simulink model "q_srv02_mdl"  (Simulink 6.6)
settings: Solver=ode1  StartTime=0.0  StopTime=inf  FixedStep=0.002  RelTol=1e-3  AbsTol=1e-6
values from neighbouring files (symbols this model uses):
  K = Am / Beq_v    [d_model_param.m]    (also in setup_srv02_exp01_mdl.m = 1)
  K_AMP = 1    [setup_srv02_exp01_mdl.m]    (also in setup_srv02_exp02_pos.m; setup_srv02_exp03_spd.m)
  K_ENC = 0    [config_srv02.m]
  K_POT = -(352 * pi / 180 / 10)    (= -0.614355896702)    [config_srv02.m]
  K_TACH = -(1000 * 2 * pi / 60 / 1.5 / Kg)    [config_srv02.m]
  tau = Jeq / Beq_v    [d_model_param.m]    (also in setup_srv02_exp01_mdl.m = 0.1)
  VMAX_AMP = 0    [config_srv02.m]
  VMAX_DAC = 10    [setup_srv02_exp01_mdl.m]    (also in setup_srv02_exp02_pos.m; setup_srv02_exp03_spd.m)
  wcf_e = 2 * pi * 25.0    (= 157.079632679)    [setup_srv02_exp01_mdl.m]    (also in setup_srv02_exp02_pos.m = 314.159265359; setup_srv02_exp03_spd.m = 395.840674352)
  zetaf_e = 0.9    [setup_srv02_exp01_mdl.m]    (also in setup_srv02_exp02_pos.m; setup_srv02_exp03_spd.m)
undefined symbols (not defined in the file or in its folder): HIL, qc_get_step_size
libraries: quarc_library x5, simulink x2

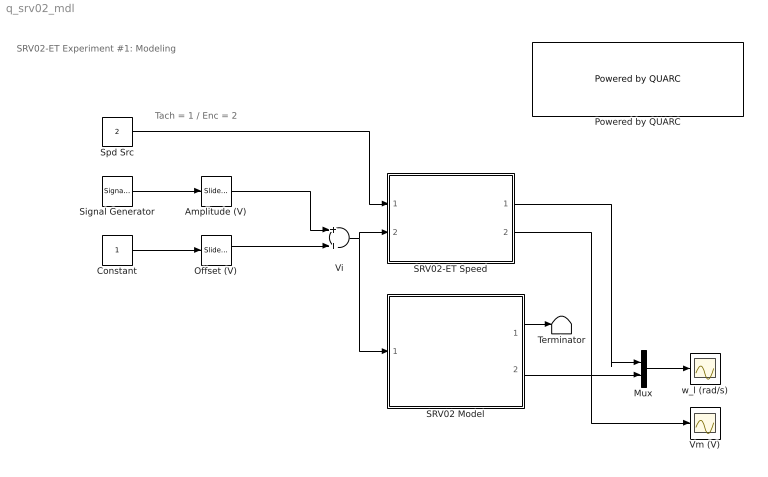
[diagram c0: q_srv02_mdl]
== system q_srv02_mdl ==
  note: SRV02-ET Experiment #1: Modeling
  note: Tach = 1 / Enc = 2
  Amplitude (V) : simulink/Math Operations/Slider Gain  SystemSampleTime=-1  low=0  gain=1  high=5
  Constant : Constant
  Mux : Mux  Inputs=2
  Offset (V) : simulink/Math Operations/Slider Gain  SystemSampleTime=-1  low=-5  gain=1.5  high=5
  Powered by QUARC : quarc_library/Logos/Powered by QUARC  SystemSampleTime=-1
  SRV02 Model : Subsystem
  SRV02-ET Speed : Subsystem
  Signal Generator : SignalGenerator  WaveForm=square  Frequency=0.4
  Spd Src : Constant  Value=2
  Terminator : Terminator
  Vi : Sum  OutScaling=2^-10
  Vm (V) : Scope
  w_l (rad/s) : Scope
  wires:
  Constant/1 -> Offset (V)/1
  Offset (V)/1 -> Vi/2
  Vi/1 -> SRV02 Model/1(Vi (V)), SRV02-ET Speed/2(Vi (V))
  Mux/1 -> w_l (rad/s)/1
  SRV02-ET Speed/2(Vm (V)) -> Vm (V)/1
  SRV02 Model/2(omega_l (rad/s)) -> Mux/2
  SRV02-ET Speed/1(omega_l (rad/s)) -> Mux/1
  SRV02 Model/1(theta_l (rad)) -> Terminator/1
  Signal Generator/1 -> Amplitude (V)/1
  Amplitude (V)/1 -> Vi/1
  Spd Src/1 -> SRV02-ET Speed/1(spd src)

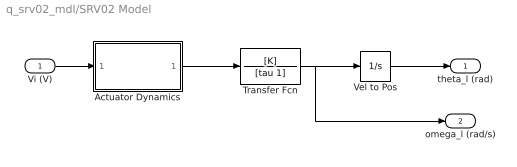
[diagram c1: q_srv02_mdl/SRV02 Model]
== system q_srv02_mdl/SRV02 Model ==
  Vi (V) : Inport
  Actuator Dynamics : Subsystem
  Transfer Fcn : TransferFcn  Numerator=[K]  Denominator=[tau 1]
  Vel to Pos : Integrator
  theta_l (rad) : Outport
  omega_l (rad/s) : Outport  Port=2
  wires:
  Vi (V)/1 -> Actuator Dynamics/1(Vi (V))
  Actuator Dynamics/1(Vm (V)) -> Transfer Fcn/1
  Vel to Pos/1 -> theta_l (rad)/1
  Transfer Fcn/1 -> Vel to Pos/1, omega_l (rad/s)/1

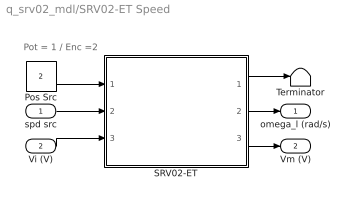
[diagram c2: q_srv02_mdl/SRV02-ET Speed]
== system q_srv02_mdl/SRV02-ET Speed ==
  note: Pot = 1 / Enc =2
  spd src : Inport
  Vi (V) : Inport  Port=2
  Pos Src : Constant  Value=2
  SRV02-ET : Subsystem
  Terminator : Terminator
  omega_l (rad/s) : Outport
  Vm (V) : Outport  Port=2
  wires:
  SRV02-ET/3(Vm (V)) -> Vm (V)/1
  Vi (V)/1 -> SRV02-ET/3(Vi (V))
  SRV02-ET/2(omega_l (rad/s)) -> omega_l (rad/s)/1
  spd src/1 -> SRV02-ET/2(spd src)
  SRV02-ET/1(theta_l (rad)) -> Terminator/1
  Pos Src/1 -> SRV02-ET/1(pos src)

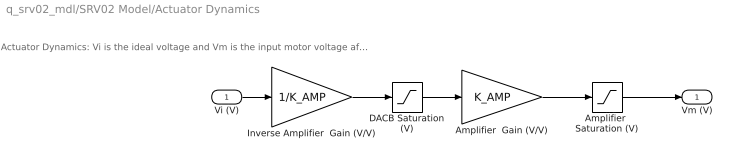
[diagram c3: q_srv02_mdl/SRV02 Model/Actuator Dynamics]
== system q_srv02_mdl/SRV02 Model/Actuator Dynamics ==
  note: Actuator Dynamics: Vi is the ideal voltage and Vm is the input motor voltage after going through the DACB and amplifier limitiations.
  Vi (V) : Inport
  Amplifier  Gain (V/V) : Gain  Gain=K_AMP
  Amplifier  Saturation (V) : Saturate  UpperLimit=VMAX_AMP  LowerLimit=-VMAX_AMP
  DACB Saturation (V) : Saturate  UpperLimit=VMAX_DAC  LowerLimit=-VMAX_DAC
  Inverse Amplifier  Gain (V/V) : Gain  Gain=1/K_AMP
  Vm (V) : Outport
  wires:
  Inverse Amplifier  Gain (V/V)/1 -> DACB Saturation (V)/1
  DACB Saturation (V)/1 -> Amplifier  Gain (V/V)/1
  Amplifier  Gain (V/V)/1 -> Amplifier  Saturation (V)/1
  Vi (V)/1 -> Inverse Amplifier  Gain (V/V)/1
  Amplifier  Saturation (V)/1 -> Vm (V)/1

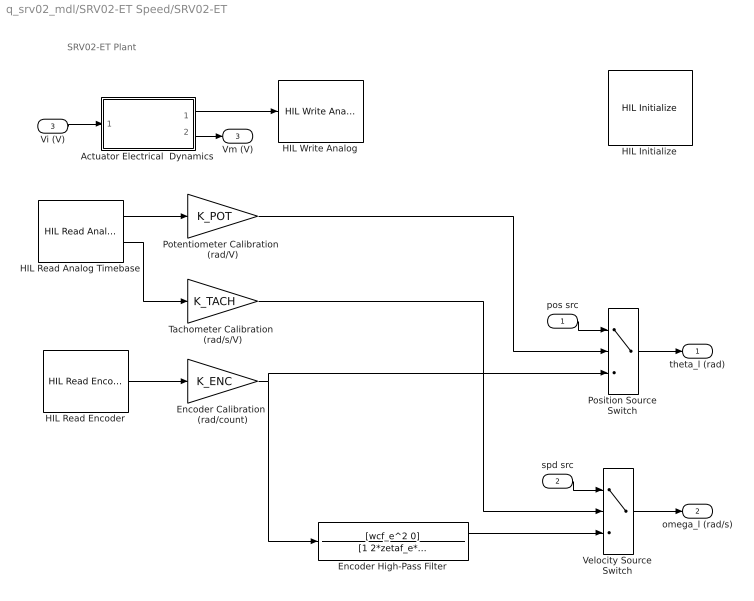
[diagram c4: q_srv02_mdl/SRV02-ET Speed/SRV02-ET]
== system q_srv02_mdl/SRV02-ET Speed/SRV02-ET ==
  note: SRV02-ET Plant
  pos src : Inport
  spd src : Inport  Port=2
  Vi (V) : Inport  Port=3
  Actuator Electrical  Dynamics : Subsystem
  Encoder Calibration  (rad/count) : Gain  Gain=K_ENC
  Encoder High-Pass Filter : TransferFcn  Numerator=[wcf_e^2 0]  Denominator=[1 2*zetaf_e*wcf_e wcf_e^2]
  HIL Initialize : quarc_library/Data Acquisition/Generic/Configuration/HIL Initialize  object_name=HIL-1  board_type=q8  board_number=0  exclusive=off  active=off  hardware_clocks=[0:1]  clock_modes=[0 0]  set_clock_params_at_start=on  set_clock_params_at_switch_in=off  analog_input_channels=[0:7]  analog_input_maximums=10  analog_input_minimums=-10  set_analog_input_params_at_start=off  set_analog_input_params_at_switch_in=off  analog_output_channels=[0:7]  analog_output_maximums=[10]  analog_output_minimums=[-10]  initial_analog_outputs=[0]  final_analog_outputs=[0]  watchdog_analog_outputs=0  set_analog_output_params_at_start=on  set_analog_output_params_at_switch_in=off  set_analog_outputs_at_start=on  set_analog_outputs_at_switch_in=off  set_analog_outputs_at_terminate=on  set_analog_outputs_at_switch_out=off  set_analog_outputs_on_watchdog=off  digital_input_channels=[]  digital_output_channels=[]  digital_output_configuration=[]  initial_digital_outputs=[1]  final_digital_outputs=[1]  watchdog_digital_outputs=[2]  set_digital_output_params_at_start=off  set_digital_output_params_at_switch_in=off  set_digital_outputs_at_start=on  set_digital_outputs_at_switch_in=off  set_digital_outputs_at_terminate=on  set_digital_outputs_at_switch_out=off  set_digital_outputs_on_watchdog=off  encoder_channels=[0:7]  quadrature=[4]  encoder_filter_frequency=(1/120e-9)/1  initial_encoder_counts=[0]  set_encoder_params_at_start=on  set_encoder_params_at_switch_in=off  set_encoder_counts_at_start=on  set_encoder_counts_at_switch_in=off  pwm_channels=[]  pwm_modes=[0]  pwm_frequency=(1/60e-9)/1024  pwm_configuration=[]  pwm_alignment=[]  pwm_polarity=[]  pwm_leading_deadband=[]  pwm_trailing_deadband=[]  initial_pwm_outputs=[0]  final_pwm_outputs=[0]  watchdog_pwm_outputs=[]  set_pwm_params_at_start=on  set_pwm_params_at_switch_in=off  set_pwm_outputs_at_start=on  set_pwm_outputs_at_switch_in=off  set_pwm_outputs_at_terminate=on  set_pwm_outputs_at_switch_out=off  set_pwm_outputs_on_watchdog=off  other_output_channels=[]  initial_other_outputs=[]  final_other_outputs=[]  watchdog_other_outputs=[]  set_other_outputs_at_start=off  set_other_outputs_at_switch_in=off  set_other_outputs_at_terminate=off  set_other_outputs_at_switch_out=off  set_other_outputs_on_watchdog=off
  HIL Read Analog Timebase : quarc_library/Data Acquisition/Generic/Timebases/HIL Read Analog Timebase  Tag=unassigned  object_name=HIL-1  clock=0  channels=[0,1]  samples_in_buffer=max(ceil(1/qc_get_step_size), 1)  active=on  vector_output=off
  HIL Read Encoder : quarc_library/Data Acquisition/Generic/Immediate I//O/HIL Read Encoder  Tag=unassigned  object_name=HIL-1  channels=0  sample_time=qc_get_step_size  active=on  vector_output=off  data_type_mode=Inherit via back propagation  data_type=double
  HIL Write Analog : quarc_library/Data Acquisition/Generic/Immediate I//O/HIL Write Analog  Tag=unassigned  object_name=HIL-1  channels=0  sample_time=-1  active=off  vector_input=off
  Position Source Switch : MultiPortSwitch  Inputs=2
  Potentiometer Calibration  (rad/V) : Gain  Gain=K_POT
  Tachometer Calibration  (rad/s/V) : Gain  Gain=K_TACH
  Velocity Source Switch : MultiPortSwitch  Inputs=2
  theta_l (rad) : Outport  InitialOutput=0
  omega_l (rad/s) : Outport  Port=2  InitialOutput=0
  Vm (V) : Outport  Port=3  InitialOutput=0
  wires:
  HIL Read Analog Timebase/2 -> Tachometer Calibration  (rad/s/V)/1
  HIL Read Encoder/1 -> Encoder Calibration  (rad/count)/1
  Encoder High-Pass Filter/1 -> Velocity Source Switch/3
  Potentiometer Calibration  (rad/V)/1 -> Position Source Switch/2
  spd src/1 -> Velocity Source Switch/1
  pos src/1 -> Position Source Switch/1
  Position Source Switch/1 -> theta_l (rad)/1
  Velocity Source Switch/1 -> omega_l (rad/s)/1
  Actuator Electrical  Dynamics/2(Vm (V)) -> Vm (V)/1
  Actuator Electrical  Dynamics/1(Vdaq (V)) -> HIL Write Analog/1
  HIL Read Analog Timebase/1 -> Potentiometer Calibration  (rad/V)/1
  Vi (V)/1 -> Actuator Electrical  Dynamics/1(Vi (V))
  Encoder Calibration  (rad/count)/1 -> Encoder High-Pass Filter/1, Position Source Switch/3
  Tachometer Calibration  (rad/s/V)/1 -> Velocity Source Switch/2

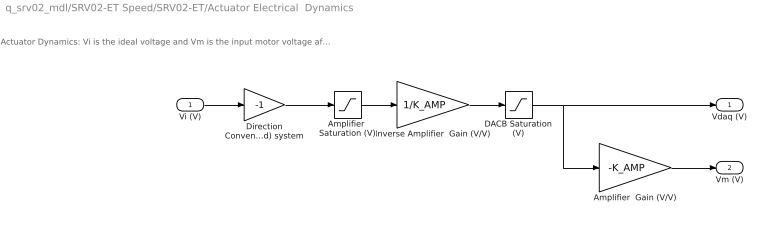
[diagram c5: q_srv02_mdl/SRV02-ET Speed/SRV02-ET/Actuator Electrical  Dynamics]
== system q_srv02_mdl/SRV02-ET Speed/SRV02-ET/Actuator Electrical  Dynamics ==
  note: Actuator Dynamics: Vi is the ideal voltage and Vm is the input motor voltage after going through the DAC and amplifier limitiations.
  Vi (V) : Inport
  Amplifier  Gain (V/V) : Gain  Gain=-K_AMP
  Amplifier  Saturation (V) : Saturate  UpperLimit=VMAX_AMP  LowerLimit=-VMAX_AMP
  DACB Saturation (V) : Saturate  UpperLimit=VMAX_DAC  LowerLimit=-VMAX_DAC
  Direction Convention: (Right-Hand) system : Gain  Gain=-1
  Inverse Amplifier  Gain (V/V) : Gain  Gain=1/K_AMP
  Vdaq (V) : Outport
  Vm (V) : Outport  Port=2
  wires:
  Vi (V)/1 -> Direction Convention: (Right-Hand) system/1
  Amplifier  Saturation (V)/1 -> Inverse Amplifier  Gain (V/V)/1
  Inverse Amplifier  Gain (V/V)/1 -> DACB Saturation (V)/1
  DACB Saturation (V)/1 -> Amplifier  Gain (V/V)/1, Vdaq (V)/1
  Amplifier  Gain (V/V)/1 -> Vm (V)/1
  Direction Convention: (Right-Hand) system/1 -> Amplifier  Saturation (V)/1
